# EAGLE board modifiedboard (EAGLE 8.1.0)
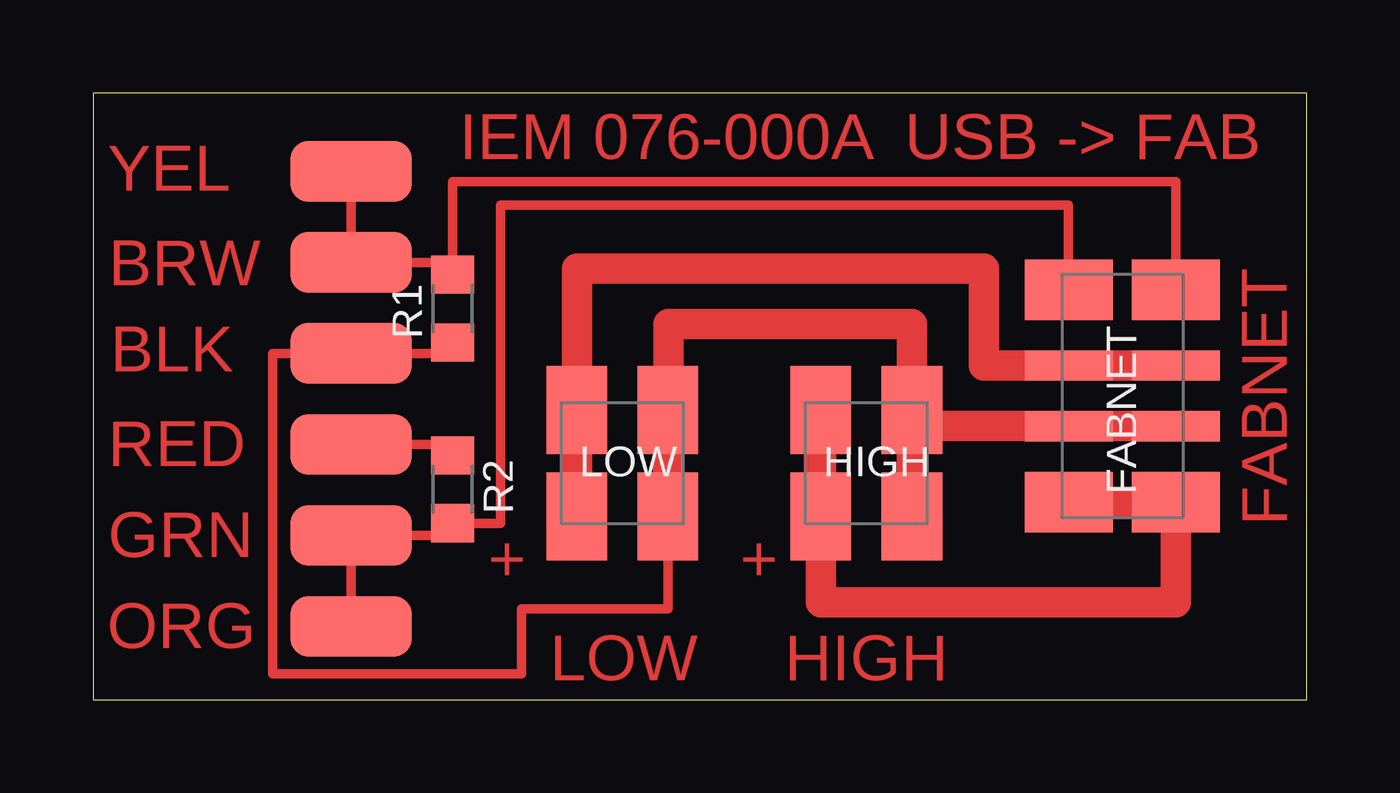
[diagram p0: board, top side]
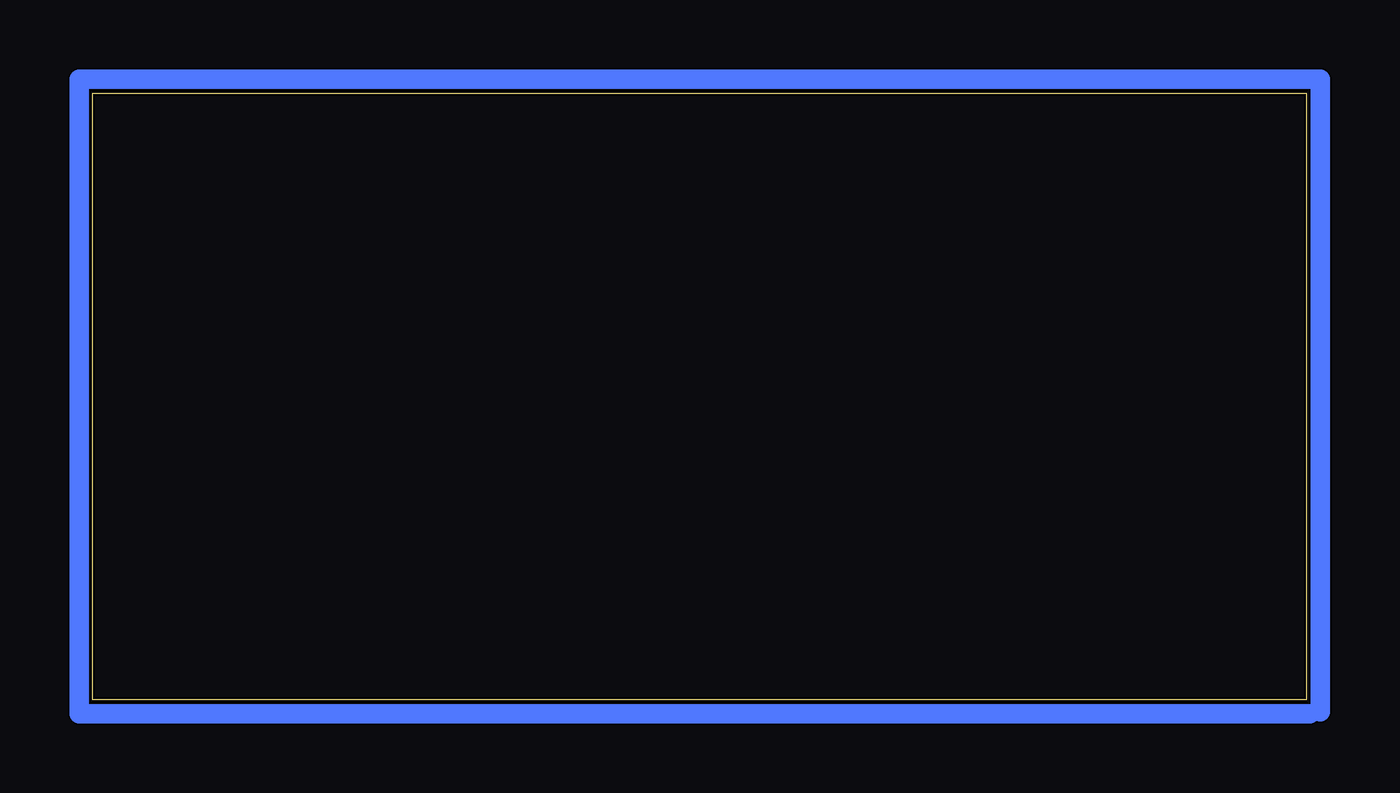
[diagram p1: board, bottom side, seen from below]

Size 50.8 x 25.4 mm. Coordinates in mm from the lower left corner, seen from the top.
Outline: 0,0 50.8,0 50.8,25.4 0,25.4 0,0
Copper layers (1*16): Top 0.035mm / dielectric 1.5mm / Bottom 0.035mm
Design rules "default": minimum track width 10mil, minimum drill 24mil, track to track 8mil, track to pad 8mil, pad to pad 8mil, via to via 8mil, smd to smd 8mil, copper to edge 40mil, drill to drill 8mil, minimum pad ring 10mil, minimum via ring 8mil, stop-mask expansion 4mil, vias tented up to drill 0mil, thermal gap 10mil

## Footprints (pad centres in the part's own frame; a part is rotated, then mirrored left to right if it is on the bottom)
IO_HEADER = smd 2.54 x 3.683: 1 -3.175,-2.235; 2 -3.175,2.235; 7 5.715,-2.235; 8 5.715,2.235 | smd 1.27 x 3.683: 3 0,-2.235; 4 0,2.235; 5 2.54,-2.235; 6 2.54,2.235
2X2HEADER = smd 2.54 x 3.683: 1 -1.905,-2.235; 2 -1.905,2.235; 3 1.905,-2.235; 4 1.905,2.235
R1206 = smd 1.6 x 1.803: 1 -1.422,0; 2 1.422,0
FABNET_PADS = smd 5.08 x 2.54: BLACK 0,2.54; BROWN 0,6.35; GREEN 0,-5.08; ORANGE 0,-8.89; RED 0,-1.27; YELLOW 0,10.16

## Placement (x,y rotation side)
FABNET  IO_HEADER  [IO_HEADER]  43.08,14 270 top
HIGH  DC_MOTOR_HEADER  [2X2HEADER]  32.36,9.91 0 top
LOW  DC_MOTOR_HEADER  [2X2HEADER]  22.15,9.91 0 top
R1  600  [R1206]  15.04,16.38 90 top
R2  600  [R1206]  15.04,8.81 270 top
U$4  FABNET_PADS  [FABNET_PADS]  10.79,11.96 0 top

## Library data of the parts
FABNET HIGH LOW U$4 = MtMM
R1 R2 = rcl

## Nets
N$1: FABNET.7 FABNET.8 HIGH.1 HIGH.2
N$3: FABNET.3 FABNET.4 LOW.1 LOW.2
N$4: FABNET.1 R2.2 U$4.GREEN U$4.ORANGE
N$5: R2.1 U$4.RED
N$6: FABNET.2 R1.2 U$4.BROWN U$4.YELLOW
N$7: FABNET.5 FABNET.6 HIGH.3 HIGH.4 LOW.3 LOW.4 R1.1 U$4.BLACK

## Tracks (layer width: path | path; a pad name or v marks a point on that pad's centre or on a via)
N$1
  Top 1.27: FABNET.7 FABNET.8 45.31,4.09 30.45,4.09 HIGH.1 HIGH.2
N$3
  Top 1.27: FABNET.4 FABNET.3 37.29,13.99 37.29,18.06 20.24,18.06 LOW.2 LOW.1
N$4
  Top 0.406: U$4.ORANGE U$4.GREEN 15.04,6.88 R2.2 17.04,7.39 17.04,20.7 40.82,20.7 40.82,17.17 FABNET.1
N$5
  Top 0.406: U$4.RED 15.04,10.69 R2.1
N$6
  Top 0.406: 15.04,18.31 R1.2 | U$4.YELLOW U$4.BROWN 15.04,18.31 | FABNET.2 45.31,21.69 15.04,21.69 15.04,18.31
N$7
  Top 0.406: R1.1 15.04,14.5 U$4.BLACK 7.52,14.5 7.52,1.09 17.93,1.09 17.93,3.81 24.05,3.81 LOW.3
  Top 1.27: FABNET.6 FABNET.5 34.27,11.46 HIGH.4 | 34.27,12.8 HIGH.4 | 34.27,12.8 34.27,13.34 | HIGH.4 HIGH.3 | LOW.3 LOW.4 24.08,15.72 34.27,15.72 34.27,12.8
S$1
  Bottom 0.813: -0.15,-0.58 51.36,-0.58 51.36,25.98 -0.58,25.98 -0.58,-0.51

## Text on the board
Top: IEM 076-000A | USB -> FAB | YEL | BRW | BLK | RED | FABNET | GRN | + | + | ORG | LOW | HIGH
